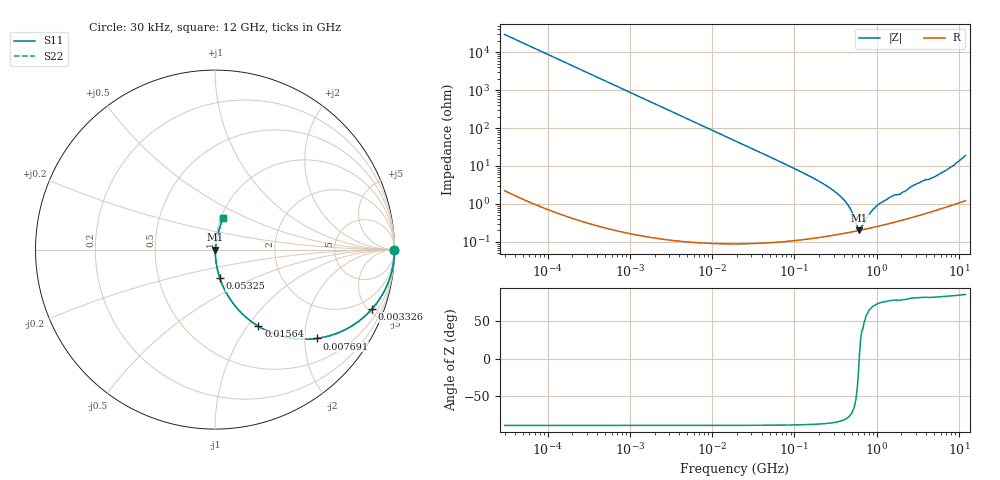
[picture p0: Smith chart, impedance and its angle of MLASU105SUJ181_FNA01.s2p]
! MLASU105SUJ181_FNA01  S-PARAMETER MODEL  ( General Type )
! Model Generated by TAIYO YUDEN Corporation (http://www.ty-top.com)
! Version 3.0
! TAIYO YUDEN Control No. 120810
! Copyright(c) 2003 TAIYO YUDEN CO.,LTD. All Rights Reserved.
! Product Description (link to TY-COMPAS)
! https://ds.yuden.co.jp/TYCOMPAS/or/detail?pn=MLASU105SUJ181JFNA01&u=M
! Products Name : Multilayer Ceramic Capacitors
! Characteristics :
!  Capacitance : 180 pF , Rated Voltage : 50V , TCC : UJ / U2J
!  Case Size : 1.0 x 0.5 / 0.039 x 0.02 [mm/inch] , Thickness : 0.5 / 0.02 [mm/inch]
!  (Conditions: Temperature = 25 degC , DC Bias Current/Voltage = 0A / 0V)
! External Node Assignments :
!  1  o---| |---o  2
! GND o---------o GND
! Frequency Range : 0.03MHz  -  12000MHz  [ 401 STEP ]
# MHz S RI R 50
! Freq[MHz].  S11 Real  S11 Imag  S21 Real  S21 Imag  S12 Real  S12 Imag  S22 Real  S22 Imag
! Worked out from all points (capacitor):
!   401 points, 30 kHz to 12 GHz, reference 50 ohm
!   read as one part in series: C = 180 pF near 32 kHz
!   lowest |Z| = 201 mohm at 617.6 MHz (marker M1)
!   series resonance near 614.9 MHz, so ESL is about 370 pH
!   S11 on the Smith chart (normalised r, x): 30 kHz: open; 3.326 MHz: 1.00, -5.31; 7.691 MHz: 1.00, -2.30; 15.64 MHz: 1.00, -1.13; 53.25 MHz: 1.00, -0.33; 12 GHz: 1.02, +0.38
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0.03  1 -0.0034  1.18e-05 0.0034  1.18e-05 0.0034  1 -0.0034
0.260295  0.9991 -0.0294  0.000871 0.0294  0.000871 0.0294  0.9991 -0.0294
0.886466  0.99 -0.0994  0.00999 0.0994  0.00999 0.0994  0.99 -0.0994
2.258455  0.9386 -0.24  0.0614 0.24  0.0614 0.24  0.9386 -0.24
3.325624  0.8757 -0.3297  0.1243 0.3297  0.1243 0.3297  0.8757 -0.3297
7.691429  0.5686 -0.4949  0.4314 0.4949  0.4314 0.4949  0.5686 -0.4949
15.63581  0.242 -0.4275  0.758 0.4275  0.758 0.4275  0.242 -0.4275
18.97367  0.1783 -0.3818  0.8217 0.3818  0.8217 0.3818  0.1783 -0.3818
29.80049  0.0811 -0.2715  0.9189 0.2715  0.9189 0.2715  0.0811 -0.2715
53.24956  0.0273 -0.16  0.9727 0.16  0.9727 0.16  0.0273 -0.16
164.6252  0.00369 -0.0496  0.9963 0.0496  0.9963 0.0496  0.00369 -0.0496
275.7901  0.0021 -0.0255  0.9979 0.0255  0.9979 0.0255  0.0021 -0.0255
393.2198  0.00183 -0.0132  0.9982 0.0132  0.9982 0.0132  0.00183 -0.0132
477.1624  0.00185 -0.00736  0.9982 0.00736  0.9982 0.00736  0.00185 -0.00736
579.0248  0.00195 -0.00174  0.998 0.00174  0.998 0.00174  0.00195 -0.00174
617.6002  0.00201 0.000134  0.998 -0.000134  0.998 -0.000134  0.00201 0.000134
658.7456  0.00207 0.00151  0.9979 -0.00151  0.9979 -0.00151  0.00207 0.00151
799.3715  0.00228 0.00472  0.9977 -0.00472  0.9977 -0.00472  0.00228 0.00472
939.2353  0.0025 0.00729  0.9975 -0.00729  0.9975 -0.00729  0.0025 0.00729
1428.372  0.00325 0.0144  0.9968 -0.0144  0.9968 -0.0144  0.00325 0.0144
5358.614  0.00983 0.0548  0.9902 -0.0548  0.9902 -0.0548  0.00983 0.0548
12000  0.045 0.1773  0.955 -0.1773  0.955 -0.1773  0.045 0.1773
